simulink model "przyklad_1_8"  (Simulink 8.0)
settings: Solver=ode45  StartTime=0.0  StopTime=0.1  RelTol=1e-11
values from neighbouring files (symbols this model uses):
  C1 = 4.7*1.E-3    (= 0.0047)    [przykl_2_8_par.m]
  C2 = 22.0*1.E-6    (= 2.2e-05)    [przykl_2_8_par.m]
  E = 100.0    (= 100)    [przykl_2_8_par.m]
  freq = 2*pi*f    (= 314.159265359)    [przykl_2_8_par.m]
  J = 5.0    (= 5)    [przykl_2_8_par.m]
  L = 2.5    [przykl_2_8_par.m]
  R1 = 10.0    (= 10)    [przykl_2_8_par.m]
  R2 = 500.0    (= 500)    [przykl_2_8_par.m]

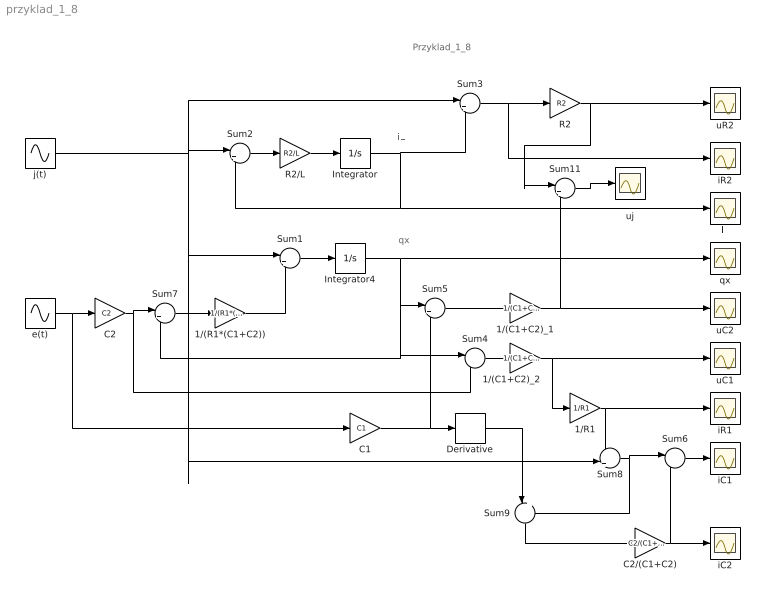
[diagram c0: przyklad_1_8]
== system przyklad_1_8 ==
  note: qx
  note: iL
  note: Przyklad_1_8
  1/(C1+C2)_1 : Gain  Gain=1/(C1+C2)
  1/(C1+C2)_2 : Gain  Gain=1/(C1+C2)
  1/(R1*(C1+C2)) : Gain  Gain=1/(R1*(C1+C2))
  1/R1 : Gain  Gain=1/R1
  C1 : Gain  Gain=C1
  C2 : Gain  Gain=C2
  C2/(C1+C2) : Gain  Gain=C2/(C1+C2)
  Derivative : Derivative
  Integrator : Integrator
  Integrator4 : Integrator
  R2 : Gain  Gain=R2
  R2/L : Gain  Gain=R2/L
  Sum{1,5,9,11} (4 alike) : Sum  Inputs=|++
  Sum2 : Sum  Inputs=|+-
  Sum3 : Sum  Inputs=|+-
  Sum4 : Sum  Inputs=|-+
  Sum6 : Sum  Inputs=|-+
  Sum7 : Sum  Inputs=|+-
  Sum8 : Sum  Inputs=+|+
  e(t) : Sin  Amplitude=E  Frequency=freq  Phase=pi  SampleTime=0
  iC1 : Scope
  iC2 : Scope
  iL : Scope
  iR1 : Scope
  iR2 : Scope
  j(t) : Sin  Amplitude=J  Frequency=freq  SampleTime=0
  qx : Scope
  uC1 : Scope
  uC2 : Scope
  uR2 : Scope
  uj : Scope
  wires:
  Sum2/1 -> R2/L/1
  Sum1/1 -> Integrator4/1
  Integrator4/1 -> Sum7/2, Sum4/1, Sum5/1, qx/1
  Integrator/1 -> iL/1, Sum2/2, Sum3/2
  1/(R1*(C1+C2))/1 -> Sum1/2
  j(t)/1 -> Sum8/2, Sum1/1, Sum2/1, Sum3/1
  Sum3/1 -> iR2/1, R2/1
  Sum4/1 -> 1/(C1+C2)_2/1
  Sum5/1 -> 1/(C1+C2)_1/1
  1/(C1+C2)_1/1 -> Sum11/2, uC2/1
  1/(C1+C2)_2/1 -> 1/R1/1, uC1/1
  1/R1/1 -> Sum8/1, iR1/1
  C2/1 -> Sum4/2, Sum7/1
  C1/1 -> Sum5/2, Derivative/1
  Derivative/1 -> Sum9/1
  C2/(C1+C2)/1 -> iC2/1, Sum6/2
  R2/L/1 -> Integrator/1
  R2/1 -> Sum11/1, uR2/1
  Sum7/1 -> 1/(R1*(C1+C2))/1
  Sum8/1 -> Sum9/2, Sum6/1
  Sum9/1 -> C2/(C1+C2)/1
  Sum6/1 -> iC1/1
  e(t)/1 -> C1/1, C2/1
  Sum11/1 -> uj/1
